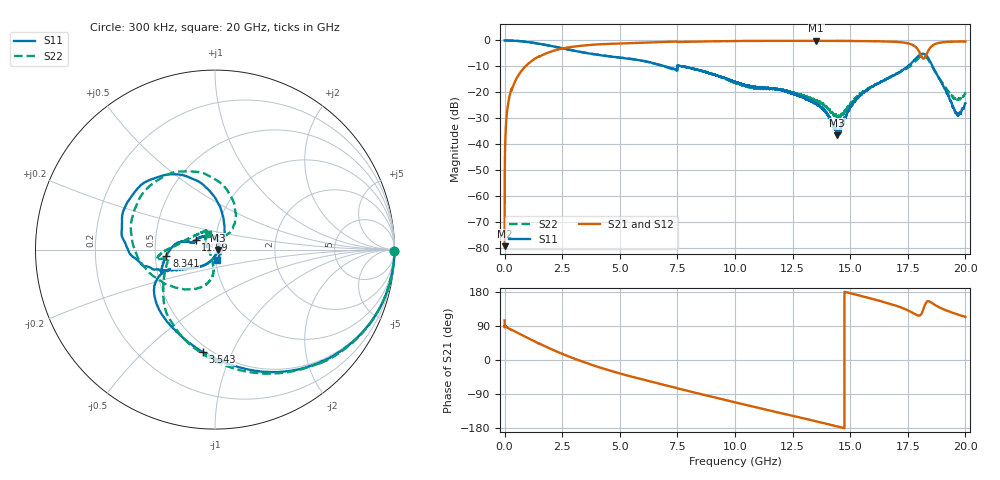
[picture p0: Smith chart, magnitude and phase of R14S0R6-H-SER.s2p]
!{R14S0R6}
!Johanson Technology Inc.
!www.johansontechnology.com
!Test Board Conditions:
!Substrate Type  RO4350B
!Substrate Thickness  20 mil
!Substrate Dk  3.66
!TL Type: GCPW
!TL Trace Width  36 mil
!TL Gap  12 mil
!Electrode orientation  Horizontal
!DUT TOPOLOGY	SERIES
!Mounting Pad LxW  26x36 mil
! Created Wed Nov 25 17:33:21 2020
! 2 Port Network Data from SP1.SP block
! freq  magS11  angS11  magS21  angS21  magS12  angS12  magS22  angS22
# khz S ma R 50
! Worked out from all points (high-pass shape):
!   20001 points, 300 kHz to 20 GHz, reference 50 ohm
!   highest |S21| = -0.13 dB at 13.52 GHz (marker M1); lowest = -79.3 dB at 300 kHz (marker M2)
!   |S21| within 3 dB of the highest: 2.504 GHz to 17.9 GHz (15.4 GHz wide, 151 % of centre); 18.45 GHz to end of sweep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
!   lowest |S11| = -36.5 dB at 14.43 GHz (marker M3), VSWR 1.03, Z = 51.5 - j0.204 ohm
!   |S11| at or under -10 dB: 6.966 GHz to 7.5 GHz (534.4 MHz wide, 7.39 % of centre); 7.722 GHz to 17.48 GHz (9.761 GHz wide, 77.5 % of centre); 18.58 GHz to end of sweep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
!   |S22| runs from -30.0 to 0.0 dB; largest |S21 - S12| = 0.014
!   S11 on the Smith chart (normalised r, x): 300 kHz: open; 3.543 GHz: 0.46, -0.78; 8.341 GHz: 0.57, -0.04; 11.59 GHz: 0.80, +0.09; 20 GHz: 1.01, -0.12
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300  0.9993 -0.4  0.0001083 104.4  0.0001631 63.4  1 -0.3
101300  0.9986 -3.6  0.03995 86.2  0.04026 86.1  0.9991 -3.5
134300  0.9982 -4.6  0.0529 85.1  0.05325 84.9  0.9982 -4.6
516300  0.9818 -16.3  0.1844 73.3  0.1848 73.4  0.9812 -16.3
1768300  0.8228 -53.2  0.5543 35.9  0.5554 35.9  0.8219 -54.3
3334300  0.596 -92.1  0.7903 -3.3  0.7914 -3.4  0.5971 -94.5
3543300  0.5742 -97.0  0.8069 -7.9  0.8076 -7.9  0.5746 -98.8
6667300  0.3455 -154.4  0.9286 -61.8  0.9295 -61.7  0.3405 -147.5
8341300  0.2724 -172.8  0.9494 -87.3  0.9513 -87.2  0.2741 -179.1
1.00003e7  0.1613 164.0  0.9744 -111.7  0.974 -111.7  0.1533 154.3
1.15933e7  0.1194 153.6  0.9798 -134.5  0.978 -134.6  0.1163 116.1
1.33343e7  0.06606 91.9  0.9811 -159.1  0.9827 -159.1  0.07383 135.3
1.35183e7  0.05924 82.5  0.9851 -161.7  0.9807 -161.7  0.07009 139.2
1.44313e7  0.01493 -7.6  0.9815 -175.2  0.9788 -175.1  0.03192 -162.1
1.53373e7  0.07781 -116.1  0.9717 171.1  0.973 171.1  0.08521 -96.6
1.66673e7  0.1864 -146.4  0.9529 149.3  0.9473 149.5  0.1899 -101.9
1.77093e7  0.3868 -165.9  0.8209 124.6  0.8205 124.4  0.3508 -150.3
1.80063e7  0.525 171.5  0.5924 117.1  0.5897 118.0  0.4714 170.5
1.81943e7  0.5501 144.7  0.4458 137.2  0.4452 138.0  0.5058 134.2
1.86533e7  0.2746 88.2  0.8412 146.4  0.8417 146.5  0.2656 65.6
1.96083e7  0.03992 -3.7  0.9546 121.3  0.9588 121.5  0.07364 79.9
2e7  0.06142 -80.3  0.9561 113.7  0.953 113.7  0.09491 115.9
